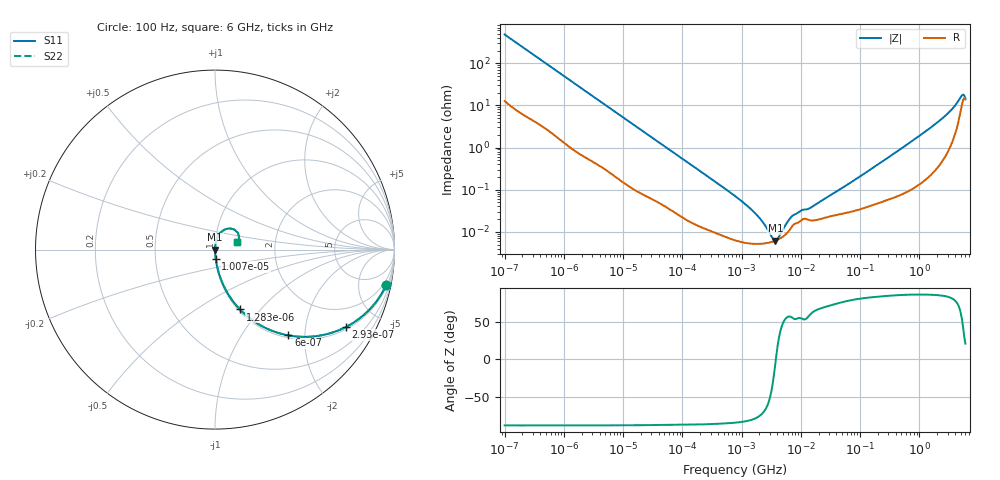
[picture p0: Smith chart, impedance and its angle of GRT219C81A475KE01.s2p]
!Murata Part Number: GRT219C81A475KE01
!These Parameters are Measured in Series Mode Connection
!Data Generated on Jun 19, 2026
!  o--ll--o
!Port1  Port2
!  o------o
!Operation Temp=25[degC], DC Bias Voltage=0[V]
!Freq. Start=100[Hz] Stop=6[GHz] 401[Steps]
# Hz S RI R 50
!Freq.(Hz) S11(Real) S11(Imag) S21(Real) S21(Imag) S12(Real) S12(Imag) S22(Real) S22(Imag)
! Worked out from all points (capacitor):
!   401 points, 100 Hz to 6 GHz, reference 50 ohm
!   read as one part in series: C = 3.29 uF near 109 Hz
!   lowest |Z| = 6.2 mohm at 3.712 MHz (marker M1)
!   series resonance near 3.796 MHz, so ESL is about 530 pH
!   S11 on the Smith chart (normalised r, x): 100 Hz: 1.25, -9.64; 293 Hz: 1.09, -3.34; 600 Hz: 1.05, -1.65; 1.283 kHz: 1.02, -0.78; 10.07 kHz: 1.00, -0.10; 6 GHz: 1.28, +0.10
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100  0.954 -0.1968  0.046 0.1968  0.046 0.1968  0.954 -0.1968
179  0.8742 -0.3194  0.1258 0.3194  0.1258 0.3194  0.8742 -0.3194
293  0.7303 -0.4306  0.2697 0.4306  0.2697 0.4306  0.7303 -0.4306
600  0.4085 -0.4779  0.5915 0.4779  0.5915 0.4779  0.4085 -0.4779
1283  0.1389 -0.3333  0.8611 0.3333  0.8611 0.3333  0.1389 -0.3333
2008  0.0648 -0.2335  0.9352 0.2335  0.9352 0.2335  0.0648 -0.2335
4111  0.0186 -0.1216  0.9814 0.1216  0.9814 0.1216  0.0186 -0.1216
10066  0.00412 -0.0514  0.9959 0.0514  0.9959 0.0514  0.00412 -0.0514
40335  0.00066 -0.0132  0.9993 0.0132  0.9993 0.0132  0.00066 -0.0132
774597  6.35e-05 -0.000705  0.9999 0.000705  0.9999 0.000705  6.35e-05 -0.000705
1658239  5.18e-05 -0.000281  0.9999 0.000281  0.9999 0.000281  5.18e-05 -0.000281
2837864  5.51e-05 -8.96e-05  0.9999 8.96e-05  0.9999 8.96e-05  5.51e-05 -8.96e-05
3712478  6.16e-05 -6.7e-06  0.9999 6.7e-06  0.9999 6.7e-06  6.16e-05 -6.7e-06
4643984  7.2e-05 6.2e-05  0.9999 -6.2e-05  0.9999 -6.2e-05  7.2e-05 6.2e-05
6644369  0.000117 0.000177  0.9999 -0.000177  0.9999 -0.000177  0.000117 0.000177
7599586  0.000149 0.000203  0.9999 -0.000203  0.9999 -0.000203  0.000149 0.000203
1.555665e7  0.000186 0.000347  0.9998 -0.000347  0.9998 -0.000347  0.000186 0.000347
3.124326e8  0.000626 0.00601  0.9994 -0.00601  0.9994 -0.00601  0.000626 0.00601
2.240541e9  0.00588 0.0438  0.9941 -0.0438  0.9941 -0.0438  0.00588 0.0438
3.8344e9  0.0245 0.0861  0.9755 -0.0861  0.9755 -0.0861  0.0245 0.0861
5.016141e9  0.0856 0.1178  0.9144 -0.1178  0.9144 -0.1178  0.0856 0.1178
6e9  0.1231 0.0398  0.8769 -0.0398  0.8769 -0.0398  0.1231 0.0398
